(* Logix 5000 AddOnInstructionDefinition export AMCI_5034_PTO_AM_MAH; software revision 37.00 *)

TYPE AMCI_5034_PTO_AM_Input_Data :
STRUCT
   ConnectionFaulted : DINT;
   MovingCW : BOOL;
   MovingCCW : BOOL;
   InHoldState : BOOL;
   Stopped : BOOL;
   AtHome : BOOL;
   Accelerating : BOOL;
   Decelerating : BOOL;
   MoveComplete : BOOL;
   HomeInvalid : BOOL;
   InvalidProfile : BOOL;
   PositionInvalid : BOOL;
   InputError : BOOL;
   CommandError : BOOL;
   ConfigurationError : BOOL;
   ModuleOK : BOOL;
   GeneralPurposeOutputStatus : BOOL;
   Input1Active : BOOL;
   Input2Active : BOOL;
   Input3Active : BOOL;
   Input4Active : BOOL;
   bit_20_reserved : BOOL;
   bit_21_reserved : BOOL;
   bit_22_reserved : BOOL;
   EncoderFollowerMode : BOOL;
   BlendMoveRunning : BOOL;
   BlendMoveAcknowledge : BOOL;
   MinimumRegistrationProgrammed : BOOL;
   EncoderMotionDirection : BOOL;
   MultipleInputsWithSameFunction : BOOL;
   FSCExceedsNumberOfDataBits : BOOL;
   AbsoluteEncoderSetupError : BOOL;
   bit_31_reserved : BOOL;
   CurrentPosition : DINT;
   EncoderPosition : DINT;
   CapturedPosition : DINT;
END_STRUCT
END_TYPE

TYPE AMCI_5034_PTO_AM_Output_Data :
STRUCT
   Command_Word : DINT;
   TargetPosition : DINT;
   TargetVelocity : UDINT;
   Acceleration : DINT;
   Deceleration : DINT;
END_STRUCT
END_TYPE

ADD_ON_INSTRUCTION AMCI_5034_PTO_AM_MAH   (* revision 1.0, vendor AMCI, ExecuteEnableInFalse *)
// AMCI Home
// Revision note:
// 10/01/2025 V1.0  Initial release of AOI
// Help:
// MOTION AXIS HOME:   Performs CW or CCW Home Moves to a Home Input.
// AXIS INPUT DATA:  Input data from the AMCI 5034-PTO-AM.   Uses the AMCI_5034_PTO_Input_Data User Defined Data Type.
// AXIS OUTPUT DATA; Output data from the AOI to the AMCI 5034-PTO-AM.    Uses the AMCI_5034_PTO_Output_Data User Defined Data Type.
// DIRECTION: 0 for Positive CW Home or  1 for Negative CCW Home
// TARGET VELOCITY: Speed of move in units of steps / sec
// ACCELERATION: Acceleration Rate in units of steps / sec / ms
// DECELERATION:  Deceleration Rate in units of steps / sec / ms
// EN (Enable) Set when rung is true, Reset when rung is false
// DN (Done) Set when command is sent to the motion device.  Reset when the rung is false.
// ER (Error) Set when a command or input error failed to clear.  Reset when the rung is false.
// IP (In Process) Set when motion is occurring.   Reset when motion stops or the rung goes false.
// PC (Process Complete) Set when the At Home Status bit is set.   Reset the next time the rung with the AOI                                      goes from false to true.
VAR_IN_OUT
   Axis_Input_Data : AMCI_5034_PTO_AM_Input_Data; {required}
   Axis_Output_Data : AMCI_5034_PTO_AM_Output_Data; {required}
END_VAR
VAR_INPUT
   Direction_0_PositiveCW_1_NegativeCCW : BOOL; {required}   // 0=home CW 1=home CCW
   TargetVelocity : DINT; {required}
   Acceleration : DINT; {required}
   Deceleration : DINT; {required}
END_VAR
VAR_OUTPUT
   EN : BOOL; {visible}   // set when rung with AOI is true
   DN : BOOL; {access Read Only, visible}   // set when move was succesfully initiated
   ER : BOOL; {visible}   // input, command, or configuration error
   IP : BOOL; {visible}   // set when motion occurring
   PC : BOOL; {visible}   // set when process complete
END_VAR
VAR
   command_data_block : DINT[5];
        [0]   // Command Bits MSW
        [1]   // Targert Position
        [2]   // Programmed Speed
        [3]   // Lower Target Position
        [4]   // Upper Programmed Speed
   motion_occurring : BOOL; {access None}
   Internal_Enable : BOOL; {access None}   // set when driver ready to receive motion command
END_VAR

ROUTINE EnableInFalse   (* ladder *)
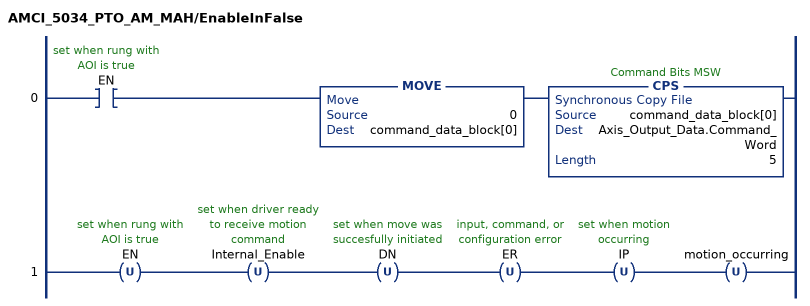
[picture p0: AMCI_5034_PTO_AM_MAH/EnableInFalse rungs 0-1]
   0: XIC(EN)MOVE(0,command_data_block[0])CPS(command_data_block[0],Axis_Output_Data.Command_Word,5);
   1: OTU(EN)OTU(Internal_Enable)OTU(DN)OTU(ER)OTU(IP)OTU(motion_occurring);
END_ROUTINE

ROUTINE Logic   (* ladder *)
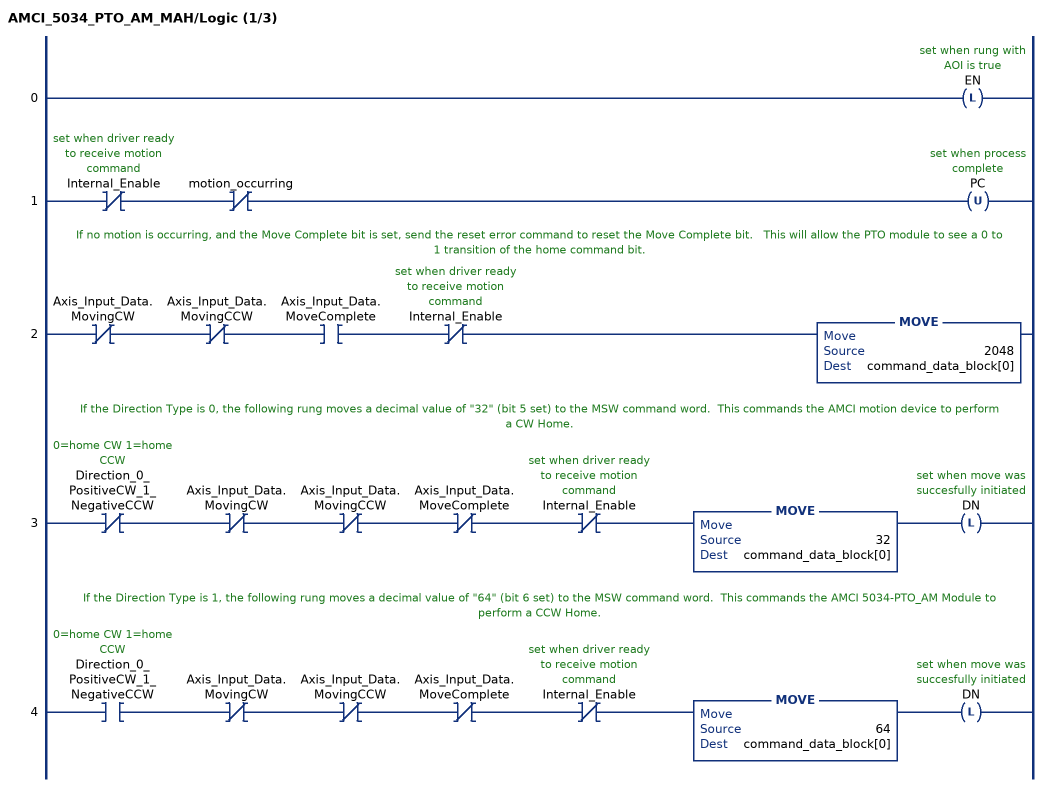
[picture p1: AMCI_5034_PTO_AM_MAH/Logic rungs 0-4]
   0: OTL(EN);
   1: XIO(Internal_Enable)XIO(motion_occurring)OTU(PC);
   // If no motion is occurring, and the Move Complete bit is set, send the reset error command to reset the Move Complete bit.   This will allow the PTO module to see a 0 to 1 transition of the home command bit.
   2: XIO(Axis_Input_Data.MovingCW)XIO(Axis_Input_Data.MovingCCW)XIC(Axis_Input_Data.MoveComplete)XIO(Internal_Enable)MOVE(2048,command_data_block[0]);
   // If the Direction Type is 0, the following rung moves a decimal value of "32" (bit 5 set) to the MSW command word.  This commands the AMCI motion device to perform a CW Home.
   3: XIO(Direction_0_PositiveCW_1_NegativeCCW)XIO(Axis_Input_Data.MovingCW)XIO(Axis_Input_Data.MovingCCW)XIO(Axis_Input_Data.MoveComplete)XIO(Internal_Enable)MOVE(32,command_data_block[0])OTL(DN);
   // If the Direction Type is 1, the following rung moves a decimal value of "64" (bit 6 set) to the MSW command word.  This commands the AMCI 5034-PTO_AM Module to perform a CCW Home.
   4: XIC(Direction_0_PositiveCW_1_NegativeCCW)XIO(Axis_Input_Data.MovingCW)XIO(Axis_Input_Data.MovingCCW)XIO(Axis_Input_Data.MoveComplete)XIO(Internal_Enable)MOVE(64,command_data_block[0])OTL(DN);
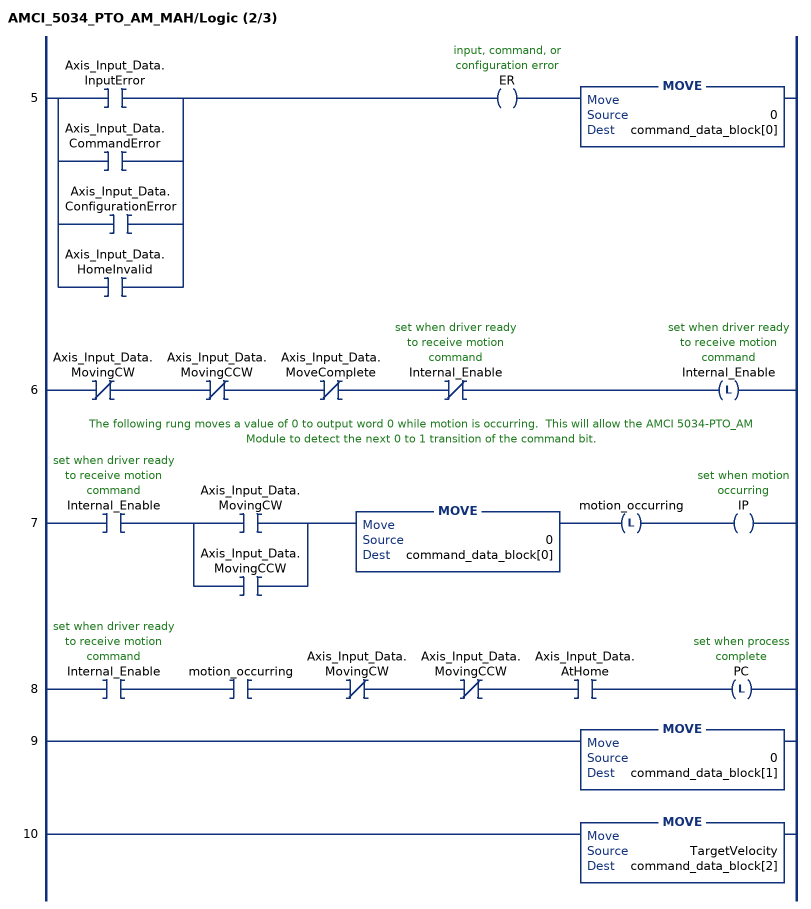
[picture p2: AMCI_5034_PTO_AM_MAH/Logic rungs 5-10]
   5: [XIC(Axis_Input_Data.InputError) ,XIC(Axis_Input_Data.CommandError) ,XIC(Axis_Input_Data.ConfigurationError) ,XIC(Axis_Input_Data.HomeInvalid) ]OTE(ER)MOVE(0,command_data_block[0]);
   6: XIO(Axis_Input_Data.MovingCW)XIO(Axis_Input_Data.MovingCCW)XIO(Axis_Input_Data.MoveComplete)XIO(Internal_Enable)OTL(Internal_Enable);
   // The following rung moves a value of 0 to output word 0 while motion is occurring.  This will allow the AMCI 5034-PTO_AM Module to detect the next 0 to 1 transition of the command bit.
   7: XIC(Internal_Enable)[XIC(Axis_Input_Data.MovingCW) ,XIC(Axis_Input_Data.MovingCCW) ]MOVE(0,command_data_block[0])OTL(motion_occurring)OTE(IP);
   8: XIC(Internal_Enable)XIC(motion_occurring)XIO(Axis_Input_Data.MovingCW)XIO(Axis_Input_Data.MovingCCW)XIC(Axis_Input_Data.AtHome)OTL(PC);
   9: MOVE(0,command_data_block[1]);
   10: MOVE(TargetVelocity,command_data_block[2]);
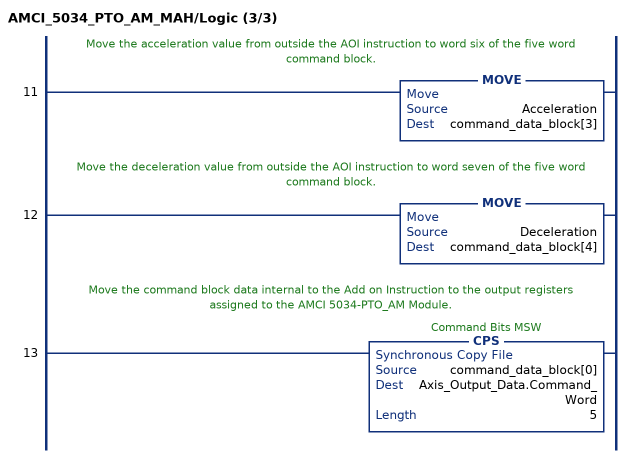
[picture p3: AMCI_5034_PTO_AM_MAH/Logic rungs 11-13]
   // Move the acceleration value from outside the AOI instruction to word six of the five word command block.
   11: MOVE(Acceleration,command_data_block[3]);
   // Move the deceleration value from outside the AOI instruction to word seven of the five word command block.
   12: MOVE(Deceleration,command_data_block[4]);
   // Move the command block data internal to the Add on Instruction to the output registers assigned to the AMCI 5034-PTO_AM Module.
   13: CPS(command_data_block[0],Axis_Output_Data.Command_Word,5);
END_ROUTINE
END_ADD_ON_INSTRUCTION
